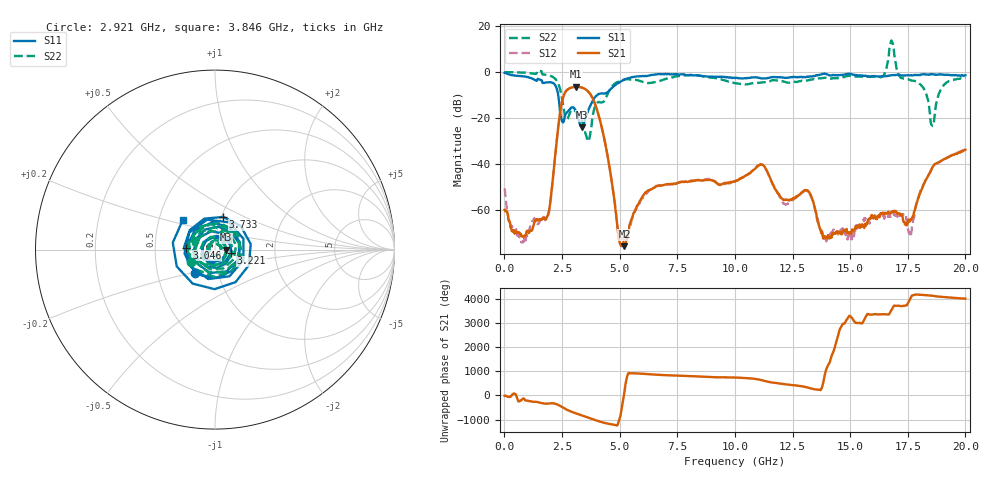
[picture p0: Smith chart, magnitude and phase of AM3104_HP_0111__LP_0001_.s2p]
!Created with skrf (http://scikit-rf.org).
# Hz S RI R 50.0
!freq ReS11 ImS11 ReS21 ImS21 ReS12 ImS12 ReS22 ImS22
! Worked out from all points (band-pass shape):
!   1601 points, 10 MHz to 20 GHz, reference 50 ohm
!   highest |S21| = -6.39 dB at 3.121 GHz (marker M1); lowest = -75.5 dB at 5.207 GHz (marker M2)
!   |S21| within 3 dB of the highest: 2.609 GHz to 3.717 GHz (1.108 GHz wide, 35 % of centre)
!   lowest |S11| = -24.0 dB at 3.346 GHz (marker M3), VSWR 1.13, Z = 56.7 - j0.129 ohm
!   |S11| at or under -10 dB: 2.335 GHz to 4.027 GHz (1.692 GHz wide, 53.2 % of centre)
!   |S22| runs from -30.0 to 13.7 dB; largest |S21 - S12| = 0.026
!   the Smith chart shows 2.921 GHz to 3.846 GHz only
!   S11 on the Smith chart (normalised r, x): 2.921 GHz: 0.78, -0.21; 3.046 GHz: 0.73, +0.02; 3.221 GHz: 1.20, -0.05; 3.733 GHz: 1.02, +0.39; 3.846 GHz: 0.66, +0.23
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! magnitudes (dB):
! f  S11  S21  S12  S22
! 10 MHz  -0.3  -59.8  -50.4  0.0
! 797.1 MHz  -1.8  -71.2  -73.9  -0.2
! 1.847 GHz  -4.5  -62.9  -63.6  -1.2
! 2.471 GHz  -20.3  -14.3  -14.4  -9.7
! 2.921 GHz  -15.4  -6.7  -6.8  -16.5
! 3.046 GHz  -16.0  -6.5  -6.5  -16.6
! 3.121 GHz  -17.2  -6.4  -6.4  -17.7
! 3.221 GHz  -20.8  -6.4  -6.5  -18.8
! 3.346 GHz  -24.0  -6.7  -6.8  -20.6
! 3.733 GHz  -14.5  -9.6  -9.7  -26.2
! 3.846 GHz  -12.3  -11.7  -11.7  -18.2
! 5.207 GHz  -3.2  -75.5  -72.0  -3.3
! 6.682 GHz  -0.9  -49.3  -49.3  -4.0
! 10.01 GHz  -2.6  -47.6  -47.5  -4.8
! 11.15 GHz  -2.8  -40.0  -40.3  -4.6
! 12.14 GHz  -2.5  -55.4  -57.0  -4.2
! 13.34 GHz  -2.0  -54.7  -55.0  -3.3
! 13.93 GHz  -0.7  -71.7  -72.2  -2.5
! 16.68 GHz  -1.5  -61.1  -62.8  7.2
! 17.6 GHz  -1.5  -64.2  -71.5  -3.4
! 18.56 GHz  -0.9  -41.4  -41.6  -23.2
! 20 GHz  -1.4  -33.7  -33.4  -2.5
